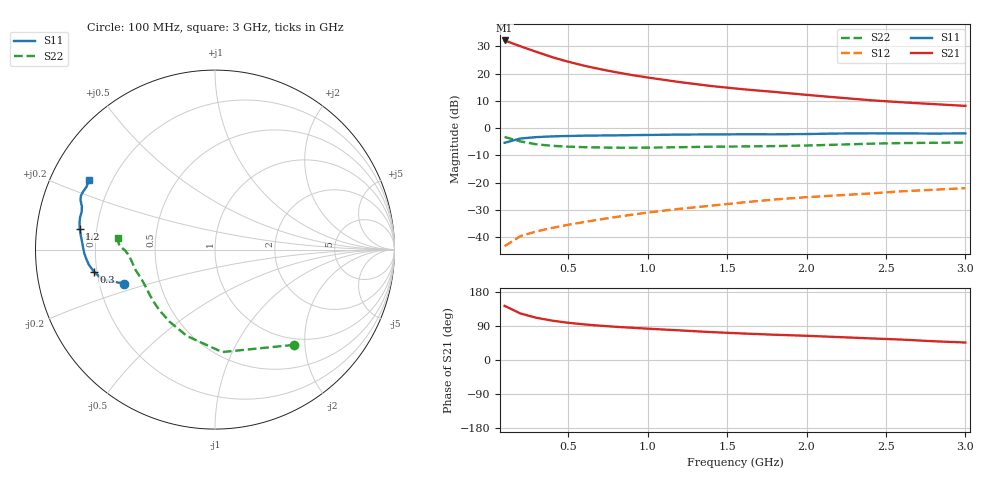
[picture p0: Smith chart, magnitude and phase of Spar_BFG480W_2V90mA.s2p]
! Filename: 290BFG480.001
! Title: BFG480W
! Bias: Vce=2V; Ic=90mA
! Company: NXP Semiconductors NL
! User: Quality&Reliability T&D
! Measure time: 10 Nov 1999 / 11:54:49
#  MHz  S  MA  R 50
! Freq  S11  S21  S12  S22  :
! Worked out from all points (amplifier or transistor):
!   20 points, 100 MHz to 3 GHz, reference 50 ohm
!   highest |S21| = 32.2 dB at 100 MHz (marker M1)
!   |S21| within 3 dB of that: start of sweep to 242.1 MHz
!   unconditionally stable (mu >= 1): 652.4 MHz to end of sweep
!   at 400 MHz: K = 0.85, MSG = 31.3 dB, |S12| = -36.5 dB
!   at 1.2 GHz: K = 1.10, MAG = 21.3 dB, |S12| = -29.6 dB
!   at 3 GHz: K = 1.10, MAG = 13.1 dB, |S12| = -22.0 dB
!   S11 on the Smith chart (normalised r, x): 100 MHz: 0.31, -0.16; 300 MHz: 0.19, -0.09; 1.2 GHz: 0.14, +0.07; 3 GHz: 0.12, +0.25
100  0.54 -159.5  40.55 142.8  0.006871 67.0  0.6888 -50.4
200  0.6463 -164.9  31.71 122.8  0.01051 58.4  0.5723 -86.0
300  0.6856 -169.6  25.04 111.4  0.01281 57.5  0.5062 -108.0
400  0.7079 -173.2  20.01 103.8  0.01489 59.5  0.4747 -122.3
500  0.7195 -176.0  16.54 98.3  0.01692 61.7  0.4585 -132.2
600  0.7285 -178.4  13.98 94.0  0.01901 63.6  0.449 -139.4
700  0.734 179.6  12.1 90.6  0.02122 65.4  0.4429 -144.8
800  0.7392 177.6  10.62 87.6  0.02353 67.3  0.4393 -149.3
900  0.745 175.8  9.436 85.1  0.02588 68.8  0.4384 -153.1
1000  0.7514 174.2  8.494 82.7  0.02836 69.8  0.4398 -156.5
1200  0.7624 171.3  7.008 78.2  0.03322 71.3  0.4479 -161.8
1400  0.7691 169.0  5.925 73.6  0.03798 72.1  0.4575 -165.8
1600  0.773 166.6  5.175 69.9  0.0435 72.7  0.4627 -169.0
1800  0.7721 164.0  4.612 66.6  0.04933 73.2  0.4696 -172.4
2000  0.7806 161.9  4.082 63.9  0.05434 73.6  0.4811 -176.1
2200  0.7983 159.8  3.638 60.5  0.05869 73.5  0.4987 -179.2
2400  0.8053 158.0  3.258 57.1  0.06352 72.9  0.519 178.8
2600  0.8026 156.3  2.982 53.9  0.06965 72.2  0.5334 177.5
2800  0.7966 153.9  2.762 49.5  0.07433 70.7  0.5393 175.7
3000  0.8016 151.3  2.565 46.1  0.07959 69.9  0.5458 173.0
